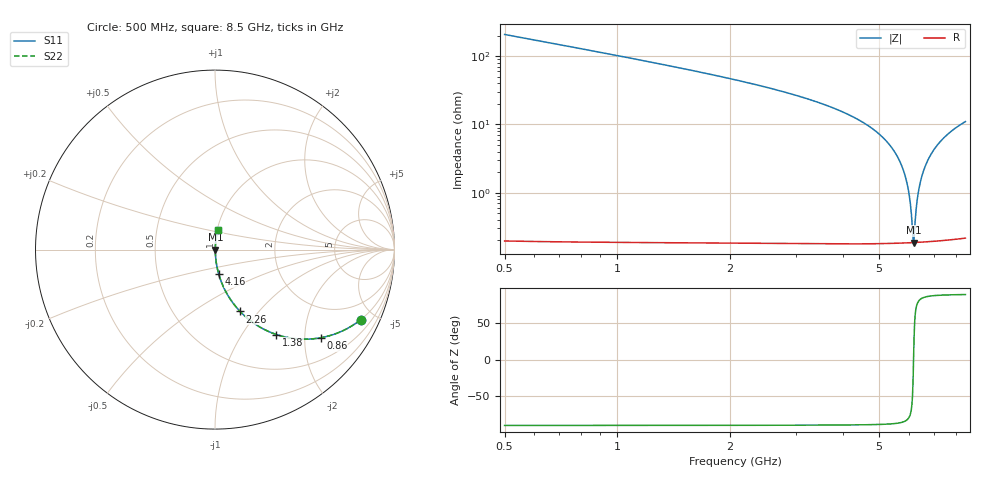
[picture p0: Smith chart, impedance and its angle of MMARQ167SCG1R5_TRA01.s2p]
! MMARQ167SCG1R5_TRA01  S-PARAMETER MODEL  ( General Type )
! Model Generated by TAIYO YUDEN Corporation (http://www.ty-top.com)
! Version 1.0
! TAIYO YUDEN Control No. 150305
! Copyright(c) 2015 TAIYO YUDEN CO.,LTD. All Rights Reserved.
! Product Description (link to TY-COMPAS)
! https://ds.yuden.co.jp/TYCOMPAS/or/detail?pn=MMARQ167SCG1R5BTRA01&u=M
! Products Name : Multilayer Ceramic Capacitors
! Characteristics :
!  Capacitance : 1.5 pF , Rated Voltage : 250V , TCC : CG / C0G
!  Case Size : 1.6 x 0.8 / 0.063 x 0.031 [mm/inch] , Thickness : 0.7 / 0.028 [mm/inch]
!  (Conditions: Temperature = 25 degC , DC Bias Current/Voltage = 0A / 0V)
! External Node Assignments :
!  1  o---| |---o  2
! GND o---------o GND
! Frequency Range : 500MHz  -  8.5GHz  [ 401 STEP ]
# MHz S RI R 50
! Freq[MHz].  S11 Real  S11 Imag  S21 Real  S21 Imag  S12 Real  S12 Imag  S22 Real  S22 Imag
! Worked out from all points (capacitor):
!   401 points, 500 MHz to 8.5 GHz, reference 50 ohm
!   read as one part in series: C = 1.52 pF near 540 MHz
!   lowest |Z| = 186 mohm at 6.18 GHz (marker M1)
!   series resonance near 6.18 GHz, so ESL is about 440 pH
!   S11 on the Smith chart (normalised r, x): 500 MHz: 1.00, -4.16; 860 MHz: 1.00, -2.39; 1.38 GHz: 1.00, -1.44; 2.26 GHz: 1.00, -0.80; 4.16 GHz: 1.00, -0.28; 8.5 GHz: 1.00, +0.22
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500  0.8122 -0.3901  0.1878 0.3901  0.1878 0.3901  0.8122 -0.3901
860  0.5878 -0.4914  0.4122 0.4914  0.4122 0.4914  0.5878 -0.4914
1380  0.3426 -0.4733  0.6574 0.4733  0.6574 0.4733  0.3426 -0.4733
1840  0.213 -0.4077  0.787 0.4077  0.787 0.4077  0.213 -0.4077
2260  0.14 -0.3448  0.86 0.3448  0.86 0.3448  0.14 -0.3448
3180  0.057 -0.2281  0.943 0.2281  0.943 0.2281  0.057 -0.2281
4160  0.0203 -0.1348  0.9797 0.1348  0.9797 0.1348  0.0203 -0.1348
4500  0.0136 -0.1078  0.9864 0.1078  0.9864 0.1078  0.0136 -0.1078
5340  0.00426 -0.0495  0.9957 0.0495  0.9957 0.0495  0.00426 -0.0495
5620  0.00285 -0.0321  0.9971 0.0321  0.9971 0.0321  0.00285 -0.0321
5840  0.0022 -0.0192  0.9978 0.0192  0.9978 0.0192  0.0022 -0.0192
6020  0.00192 -0.00888  0.9981 0.00888  0.9981 0.00888  0.00192 -0.00888
6080  0.00188 -0.00552  0.9981 0.00552  0.9981 0.00552  0.00188 -0.00552
6140  0.00186 -0.0022  0.9981 0.0022  0.9981 0.0022  0.00186 -0.0022
6180  0.00186 -6.27e-06  0.9981 6.27e-06  0.9981 6.27e-06  0.00186 -6.27e-06
6220  0.00186 0.00218  0.9981 -0.00218  0.9981 -0.00218  0.00186 0.00218
6280  0.00189 0.00542  0.9981 -0.00542  0.9981 -0.00542  0.00189 0.00542
6340  0.00194 0.00864  0.9981 -0.00864  0.9981 -0.00864  0.00194 0.00864
6500  0.00218 0.0171  0.9978 -0.0171  0.9978 -0.0171  0.00218 0.0171
6780  0.0029 0.0314  0.9971 -0.0314  0.9971 -0.0314  0.0029 0.0314
7180  0.00455 0.0508  0.9955 -0.0508  0.9955 -0.0508  0.00455 0.0508
8500  0.0141 0.1083  0.9859 -0.1083  0.9859 -0.1083  0.0141 0.1083
